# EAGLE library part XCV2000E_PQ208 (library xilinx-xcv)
xcv2000e_pq208 edit this description Auto generated by make-symbol-device-package-bsdl.ulp Rev. 26 Source: xcv2000e_pq208.bsd
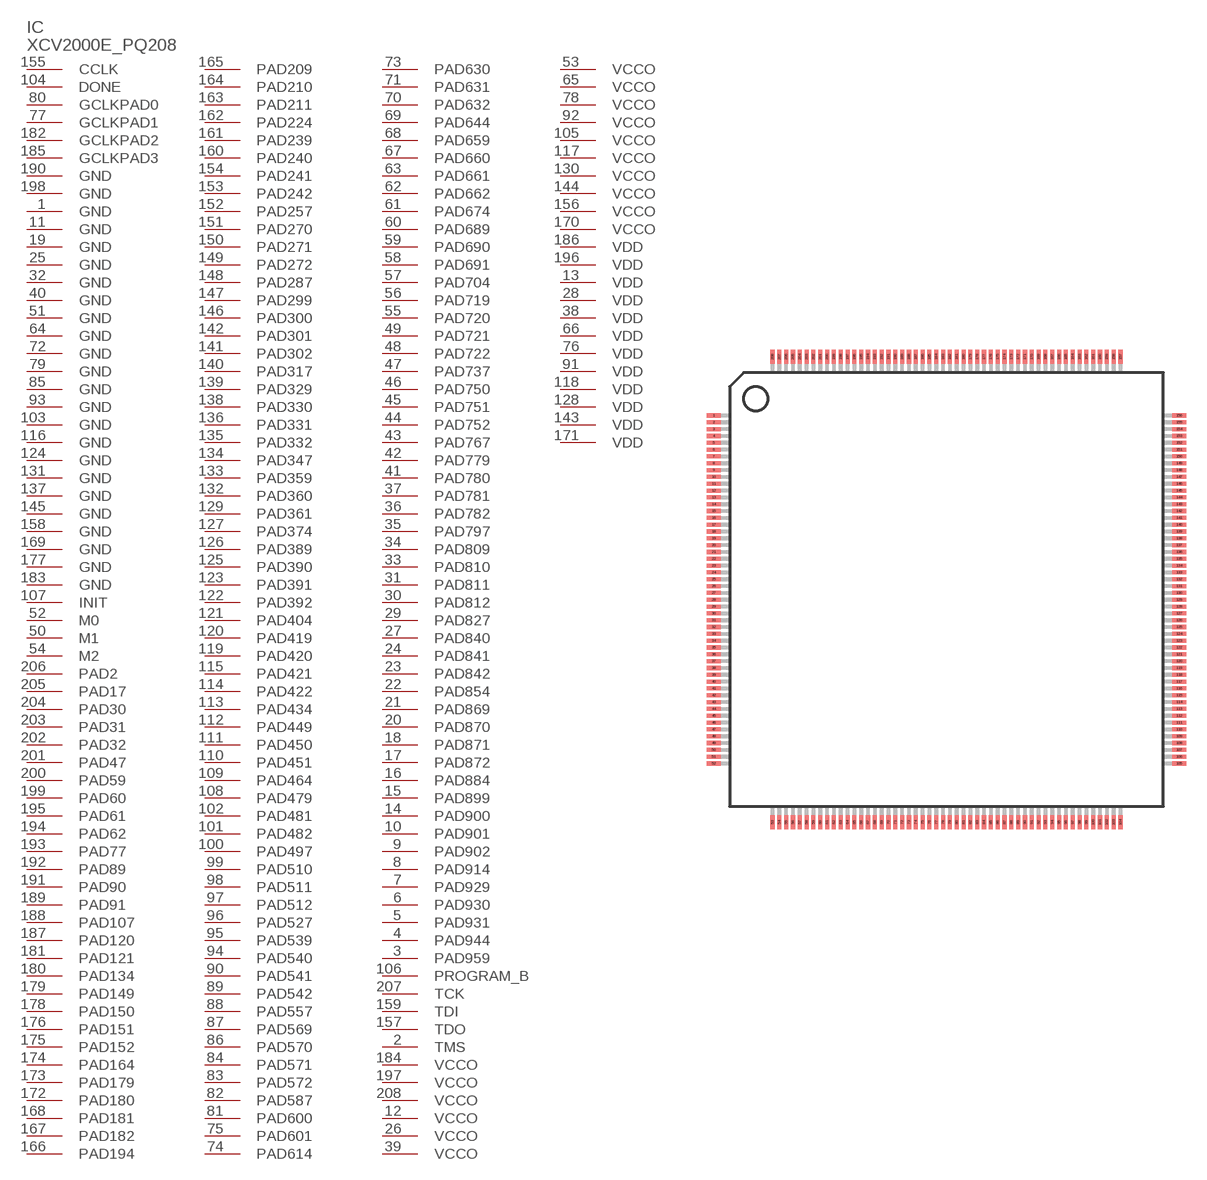
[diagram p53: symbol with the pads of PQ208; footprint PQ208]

Designator prefix IC

## XCV2000E_PQ208 (OC_FARNELL: unknown; OC_NEWARK: unknown)  [PQ208]
1  GND  pwr
2  TMS  in
3  PAD959
4  PAD944
5  PAD931
6  PAD930
7  PAD929
8  PAD914
9  PAD902
10  PAD901
11  GND  pwr
12  VCCO  pwr
13  VDD  pwr
14  PAD900
15  PAD899
16  PAD884
17  PAD872
18  PAD871
19  GND  pwr
20  PAD870
21  PAD869
22  PAD854
23  PAD842
24  PAD841
25  GND  pwr
26  VCCO  pwr
27  PAD840
28  VDD  pwr
29  PAD827
30  PAD812
31  PAD811
32  GND  pwr
33  PAD810
34  PAD809
35  PAD797
36  PAD782
37  PAD781
38  VDD  pwr
39  VCCO  pwr
40  GND  pwr
41  PAD780
42  PAD779
43  PAD767
44  PAD752
45  PAD751
46  PAD750
47  PAD737
48  PAD722
49  PAD721
50  M1  in
51  GND  pwr
52  M0  in
53  VCCO  pwr
54  M2  in
55  PAD720
56  PAD719
57  PAD704
58  PAD691
59  PAD690
60  PAD689
61  PAD674
62  PAD662
63  PAD661
64  GND  pwr
65  VCCO  pwr
66  VDD  pwr
67  PAD660
68  PAD659
69  PAD644
70  PAD632
71  PAD631
72  GND  pwr
73  PAD630
74  PAD614
75  PAD601
76  VDD  pwr
77  GCLKPAD1  in
78  VCCO  pwr
79  GND  pwr
80  GCLKPAD0  in
81  PAD600
82  PAD587
83  PAD572
84  PAD571
85  GND  pwr
86  PAD570
87  PAD569
88  PAD557
89  PAD542
90  PAD541
91  VDD  pwr
92  VCCO  pwr
93  GND  pwr
94  PAD540
95  PAD539
96  PAD527
97  PAD512
98  PAD511
99  PAD510
100  PAD497
101  PAD482
102  PAD481
103  GND  pwr
104  DONE
105  VCCO  pwr
106  PROGRAM_B  in
107  INIT
108  PAD479
109  PAD464
110  PAD451
111  PAD450
112  PAD449
113  PAD434
114  PAD422
115  PAD421
116  GND  pwr
117  VCCO  pwr
118  VDD  pwr
119  PAD420
120  PAD419
121  PAD404
122  PAD392
123  PAD391
124  GND  pwr
125  PAD390
126  PAD389
127  PAD374
128  VDD  pwr
129  PAD361
130  VCCO  pwr
131  GND  pwr
132  PAD360
133  PAD359
134  PAD347
135  PAD332
136  PAD331
137  GND  pwr
138  PAD330
139  PAD329
140  PAD317
141  PAD302
142  PAD301
143  VDD  pwr
144  VCCO  pwr
145  GND  pwr
146  PAD300
147  PAD299
148  PAD287
149  PAD272
150  PAD271
151  PAD270
152  PAD257
153  PAD242
154  PAD241
155  CCLK
156  VCCO  pwr
157  TDO  out
158  GND  pwr
159  TDI  in
160  PAD240
161  PAD239
162  PAD224
163  PAD211
164  PAD210
165  PAD209
166  PAD194
167  PAD182
168  PAD181
169  GND  pwr
170  VCCO  pwr
171  VDD  pwr
172  PAD180
173  PAD179
174  PAD164
175  PAD152
176  PAD151
177  GND  pwr
178  PAD150
179  PAD149
180  PAD134
181  PAD121
182  GCLKPAD2  in
183  GND  pwr
184  VCCO  pwr
185  GCLKPAD3  in
186  VDD  pwr
187  PAD120
188  PAD107
189  PAD91
190  GND  pwr
191  PAD90
192  PAD89
193  PAD77
194  PAD62
195  PAD61
196  VDD  pwr
197  VCCO  pwr
198  GND  pwr
199  PAD60
200  PAD59
201  PAD47
202  PAD32
203  PAD31
204  PAD30
205  PAD17
206  PAD2
207  TCK  in
208  VCCO  pwr

## Footprint PQ208 (pad centres in mm)
PQ208 Auto generated by make-symbol-device-package-bsdl.ulp Rev. 26
smd 1 x 0.3: 1 -17.05,12.75; 2 -17.05,12.25; 3 -17.05,11.75; 4 -17.05,11.25; 5 -17.05,10.75; 6 -17.05,10.25; 7 -17.05,9.75; 8 -17.05,9.25; 9 -17.05,8.75; 10 -17.05,8.25; 11 -17.05,7.75; 12 -17.05,7.25; 13 -17.05,6.75; 14 -17.05,6.25; 15 -17.05,5.75; 16 -17.05,5.25; 17 -17.05,4.75; 18 -17.05,4.25; 19 -17.05,3.75; 20 -17.05,3.25; 21 -17.05,2.75; 22 -17.05,2.25; 23 -17.05,1.75; 24 -17.05,1.25; 25 -17.05,0.75; 26 -17.05,0.25; 27 -17.05,-0.25; 28 -17.05,-0.75; 29 -17.05,-1.25; 30 -17.05,-1.75; 31 -17.05,-2.25; 32 -17.05,-2.75; 33 -17.05,-3.25; 34 -17.05,-3.75; 35 -17.05,-4.25; 36 -17.05,-4.75; 37 -17.05,-5.25; 38 -17.05,-5.75; 39 -17.05,-6.25; 40 -17.05,-6.75; 41 -17.05,-7.25; 42 -17.05,-7.75; 43 -17.05,-8.25; 44 -17.05,-8.75; 45 -17.05,-9.25; 46 -17.05,-9.75; 47 -17.05,-10.25; 48 -17.05,-10.75; 49 -17.05,-11.25; 50 -17.05,-11.75; 51 -17.05,-12.25; 52 -17.05,-12.75; 105 17.05,-12.75; 106 17.05,-12.25; 107 17.05,-11.75; 108 17.05,-11.25; 109 17.05,-10.75; 110 17.05,-10.25; 111 17.05,-9.75; 112 17.05,-9.25; 113 17.05,-8.75; 114 17.05,-8.25; 115 17.05,-7.75; 116 17.05,-7.25; 117 17.05,-6.75; 118 17.05,-6.25; 119 17.05,-5.75; 120 17.05,-5.25; 121 17.05,-4.75; 122 17.05,-4.25; 123 17.05,-3.75; 124 17.05,-3.25; 125 17.05,-2.75; 126 17.05,-2.25; 127 17.05,-1.75; 128 17.05,-1.25; 129 17.05,-0.75; 130 17.05,-0.25; 131 17.05,0.25; 132 17.05,0.75; 133 17.05,1.25; 134 17.05,1.75; 135 17.05,2.25; 136 17.05,2.75; 137 17.05,3.25; 138 17.05,3.75; 139 17.05,4.25; 140 17.05,4.75; 141 17.05,5.25; 142 17.05,5.75; 143 17.05,6.25; 144 17.05,6.75; 145 17.05,7.25; 146 17.05,7.75; 147 17.05,8.25; 148 17.05,8.75; 149 17.05,9.25; 150 17.05,9.75; 151 17.05,10.25; 152 17.05,10.75; 153 17.05,11.25; 154 17.05,11.75; 155 17.05,12.25; 156 17.05,12.75
smd 0.3 x 1: 53 -12.75,-17.05; 54 -12.25,-17.05; 55 -11.75,-17.05; 56 -11.25,-17.05; 57 -10.75,-17.05; 58 -10.25,-17.05; 59 -9.75,-17.05; 60 -9.25,-17.05; 61 -8.75,-17.05; 62 -8.25,-17.05; 63 -7.75,-17.05; 64 -7.25,-17.05; 65 -6.75,-17.05; 66 -6.25,-17.05; 67 -5.75,-17.05; 68 -5.25,-17.05; 69 -4.75,-17.05; 70 -4.25,-17.05; 71 -3.75,-17.05; 72 -3.25,-17.05; 73 -2.75,-17.05; 74 -2.25,-17.05; 75 -1.75,-17.05; 76 -1.25,-17.05; 77 -0.75,-17.05; 78 -0.25,-17.05; 79 0.25,-17.05; 80 0.75,-17.05; 81 1.25,-17.05; 82 1.75,-17.05; 83 2.25,-17.05; 84 2.75,-17.05; 85 3.25,-17.05; 86 3.75,-17.05; 87 4.25,-17.05; 88 4.75,-17.05; 89 5.25,-17.05; 90 5.75,-17.05; 91 6.25,-17.05; 92 6.75,-17.05; 93 7.25,-17.05; 94 7.75,-17.05; 95 8.25,-17.05; 96 8.75,-17.05; 97 9.25,-17.05; 98 9.75,-17.05; 99 10.25,-17.05; 100 10.75,-17.05; 101 11.25,-17.05; 102 11.75,-17.05; 103 12.25,-17.05; 104 12.75,-17.05; 157 12.75,17.05; 158 12.25,17.05; 159 11.75,17.05; 160 11.25,17.05; 161 10.75,17.05; 162 10.25,17.05; 163 9.75,17.05; 164 9.25,17.05; 165 8.75,17.05; 166 8.25,17.05; 167 7.75,17.05; 168 7.25,17.05; 169 6.75,17.05; 170 6.25,17.05; 171 5.75,17.05; 172 5.25,17.05; 173 4.75,17.05; 174 4.25,17.05; 175 3.75,17.05; 176 3.25,17.05; 177 2.75,17.05; 178 2.25,17.05; 179 1.75,17.05; 180 1.25,17.05; 181 0.75,17.05; 182 0.25,17.05; 183 -0.25,17.05; 184 -0.75,17.05; 185 -1.25,17.05; 186 -1.75,17.05; 187 -2.25,17.05; 188 -2.75,17.05; 189 -3.25,17.05; 190 -3.75,17.05; 191 -4.25,17.05; 192 -4.75,17.05; 193 -5.25,17.05; 194 -5.75,17.05; 195 -6.25,17.05; 196 -6.75,17.05; 197 -7.25,17.05; 198 -7.75,17.05; 199 -8.25,17.05; 200 -8.75,17.05; 201 -9.25,17.05; 202 -9.75,17.05; 203 -10.25,17.05; 204 -10.75,17.05; 205 -11.25,17.05; 206 -11.75,17.05; 207 -12.25,17.05; 208 -12.75,17.05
